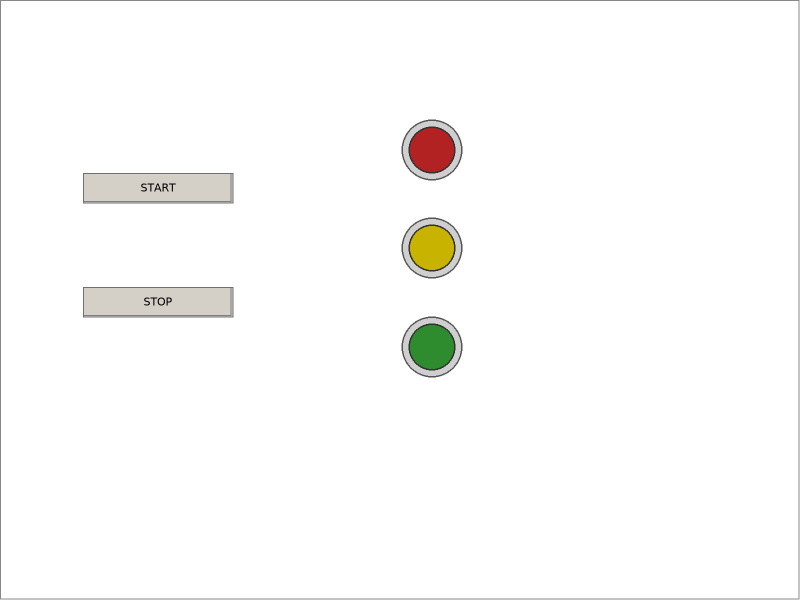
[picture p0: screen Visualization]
VISUALIZATION Visualization  // 800x600
    Button (83,173 150x30), "START"
        tap Gvl.bStart
    Button (83,287 150x30), "STOP"
        tap Gvl.bStop
    Lamp1 (397,213 70x70), variable: Gvl.Yellow, style: Lamp-Lamp1-Yellow
    Lamp1 (397,115 70x70), variable: Gvl.Red, style: Lamp-Lamp1-Red
    Lamp1 (397,312 70x70), variable: Gvl.Green, style: Lamp-Lamp1-Green
END_VISUALIZATION
